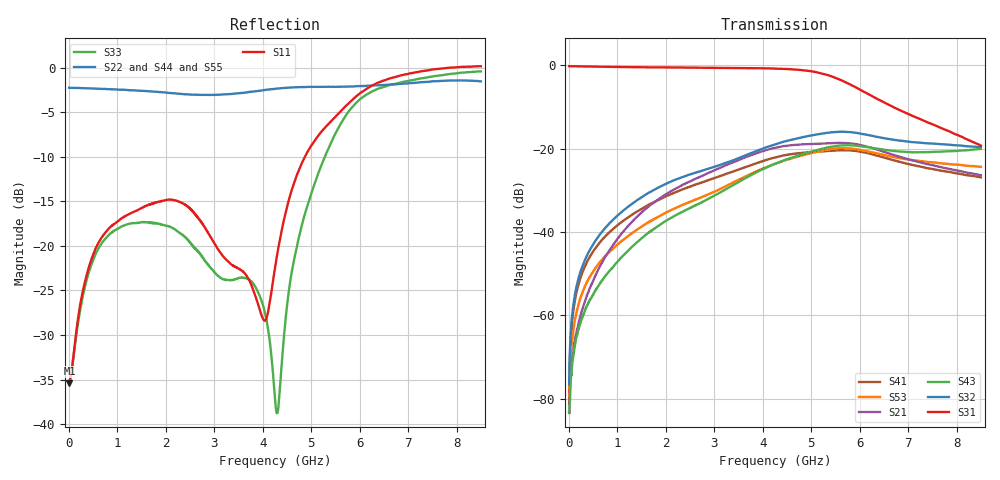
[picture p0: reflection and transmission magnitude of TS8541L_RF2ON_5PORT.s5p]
! Created with skrf (http://scikit-rf.org).
# Hz S RI R 50.0
!freq ReS11 ImS11 ReS12 ImS12 ReS13 ImS13
! ReS14 ImS14 ReS15 ImS15
! ReS21 ImS21 ReS22 ImS22 ReS23 ImS23
! ReS24 ImS24 ReS25 ImS25
! ReS31 ImS31 ReS32 ImS32 ReS33 ImS33
! ReS34 ImS34 ReS35 ImS35
! ReS41 ImS41 ReS42 ImS42 ReS43 ImS43
! ReS44 ImS44 ReS45 ImS45
! ReS51 ImS51 ReS52 ImS52 ReS53 ImS53
! ReS54 ImS54 ReS55 ImS55
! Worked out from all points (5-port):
!   1601 points, 10 MHz to 8.5 GHz, reference 50 ohm
!   strongest paths, dB at 10 MHz, 2.132 GHz, 4.255 GHz, 6.378 GHz, 8.5 GHz:
!     S31: -0.2, -0.5, -0.8, -8.1, -19.2
!     S32: -76.6, -27.7, -19.0, -17.2, -19.6
!     S43: -83.2, -36.5, -23.6, -20.0, -20.0
!     S21: -83.2, -30.0, -19.8, -20.3, -26.4
!     S53: -81.4, -34.6, -23.6, -21.1, -24.3
!     S41: -78.3, -30.8, -22.1, -21.7, -26.9
!   lowest |S11| = -35.4 dB at 15.31 MHz (marker M1), VSWR 1.03, Z = 51.7 - j0.279 ohm
!   |S11| at or under -10 dB: start of sweep to 4.871 GHz
